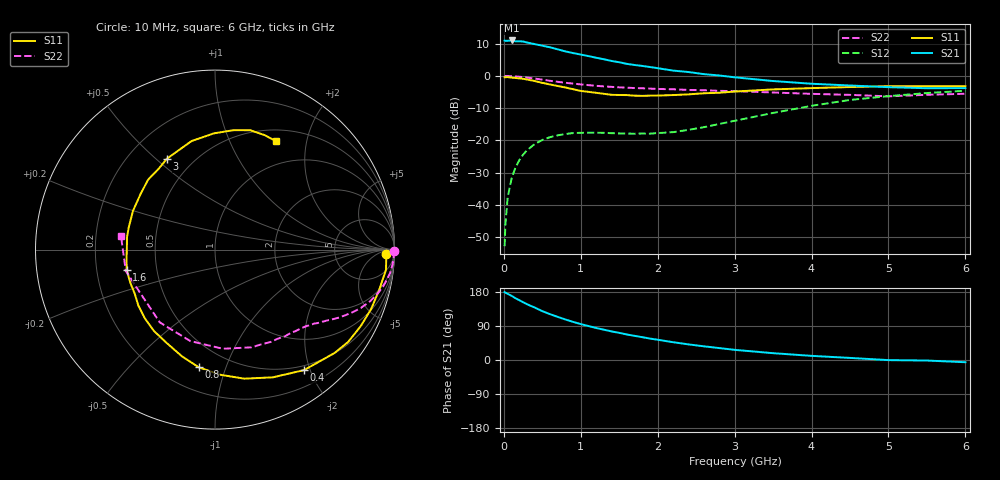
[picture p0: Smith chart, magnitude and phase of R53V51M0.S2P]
! SIEMENS Small Signal Semiconductors
! BFR183
! Si NPN RF Bipolar Junction Transistor in SOT23
! VCE = 3.5 V  IC = 1 mA
! Common Emitter S-Parameters:  May  1996
# GHz  S  MA  R  50
!  f  S11  S21  S12  S22
! GHz  MAG  ANG  MAG  ANG  MAG  ANG  MAG  ANG
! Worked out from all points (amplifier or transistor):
!   36 points, 10 MHz to 6 GHz, reference 50 ohm
!   highest |S21| = 11.0 dB at 100 MHz (marker M1)
!   |S21| within 3 dB of that: start of sweep to 738.9 MHz
!   unconditionally stable (mu >= 1): 1.646 GHz to 2.944 GHz
!   at 250 MHz: K = 0.16, MSG = 17.5 dB, |S12| = -24.4 dB
!   at 1.4 GHz: K = 0.86, MSG = 11.2 dB, |S12| = -17.7 dB
!   at 6 GHz: K = 0.95, MSG = 0.4 dB, |S12| = -4.6 dB
!   S11 on the Smith chart (normalised r, x): 10 MHz: 32, -18; 400 MHz: 0.43, -1.91; 800 MHz: 0.35, -0.81; 1.6 GHz: 0.33, -0.10; 3 GHz: 0.36, +0.54; 6 GHz: 0.65, +1.51
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0.01  0.9536 -1.5  3.528 179.3  0.0023 86.2  0.9993 -0.5
0.02  0.9553 -2.8  3.498 177.7  0.0049 87.9  0.9949 -1.0
0.05  0.9593 -6.8  3.504 174.6  0.0131 86.0  0.9963 -2.6
0.1  0.9413 -14.0  3.548 169.4  0.0256 82.2  0.9919 -5.1
0.15  0.9308 -20.9  3.445 163.2  0.0378 77.1  0.9836 -7.7
0.25  0.9028 -34.7  3.421 152.6  0.0603 69.2  0.9587 -12.4
0.3  0.8809 -40.8  3.301 147.3  0.0703 66.0  0.9423 -14.6
0.4  0.835 -53.5  3.117 138.5  0.0879 59.2  0.912 -18.3
0.5  0.7814 -65.6  2.942 128.9  0.1017 52.9  0.8764 -21.7
0.6  0.7374 -77.2  2.78 121.0  0.1126 47.8  0.8411 -24.6
0.8  0.6623 -97.8  2.401 106.9  0.1259 39.5  0.7837 -29.0
0.9  0.6225 -107.2  2.26 100.6  0.1302 36.8  0.7607 -30.7
1.1  0.5668 -126.9  2.029 89.6  0.1321 32.8  0.7197 -34.0
1.3  0.5286 -143.9  1.814 80.0  0.1316 30.8  0.6887 -36.8
1.6  0.5048 -167.0  1.538 67.3  0.128 31.7  0.6576 -41.0
1.9  0.4951 171.9  1.375 56.6  0.1276 37.3  0.6365 -45.8
2.2  0.5055 154.6  1.21 47.0  0.1345 44.3  0.6216 -50.8
3  0.5729 117.9  0.953 26.8  0.2019 57.3  0.5814 -69.5
3.5  0.6187 102.2  0.834 18.0  0.2671 56.2  0.5541 -85.5
4.5  0.6732 81.2  0.711 5.5  0.4244 43.0  0.5091 -127.1
5.5  0.6951 66.3  0.645 -1.4  0.5434 25.9  0.5108 -166.6
6  0.6929 60.7  0.648 -5.9  0.5895 15.7  0.5293 171.8
